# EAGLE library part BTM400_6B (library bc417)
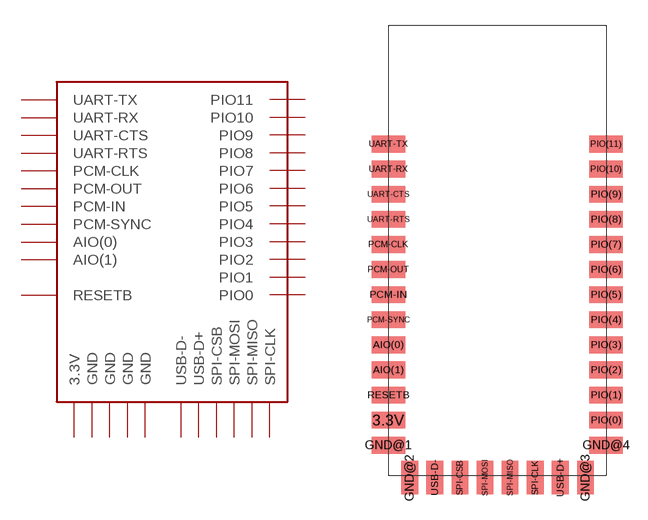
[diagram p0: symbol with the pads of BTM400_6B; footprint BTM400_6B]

Designator prefix -

## BTM400_6B  [BTM400_6B]
3.3V  3.3V  pwr
AIO(0)  AIO(0)
AIO(1)  AIO(1)
GND@1  GND  pwr
GND@2  GND  pwr
GND@3  GND  pwr
GND@4  GND  pwr
PCM-CLK  PCM-CLK
PCM-IN  PCM-IN
PCM-OUT  PCM-OUT
PCM-SYNC  PCM-SYNC
PIO(0)  PIO0
PIO(1)  PIO1
PIO(2)  PIO2
PIO(3)  PIO3
PIO(4)  PIO4
PIO(5)  PIO5
PIO(6)  PIO6
PIO(7)  PIO7
PIO(8)  PIO8
PIO(9)  PIO9
PIO(10)  PIO10
PIO(11)  PIO11
RESETB  RESETB
SPI-CLK  SPI-CLK
SPI-CSB  SPI-CSB
SPI-MISO  SPI-MISO
SPI-MOSI  SPI-MOSI
UART-CTS  UART-CTS
UART-RTS  UART-RTS
UART-RX  UART-RX
UART-TX  UART-TX
USB-D+  USB-D+
USB-D-  USB-D-

## Footprint BTM400_6B (pad centres in mm)
smd 2 x 1: 3.3V -6.5,-10.16; AIO(0) -6.5,-5.66; AIO(1) -6.5,-7.16; GND@1 -6.5,-11.66; GND@4 6.5,-11.66; PCM-CLK -6.5,0.34; PCM-IN -6.5,-2.66; PCM-OUT -6.5,-1.16; PCM-SYNC -6.5,-4.16; PIO(0) 6.5,-10.16; PIO(1) 6.5,-8.66; PIO(2) 6.5,-7.16; PIO(3) 6.5,-5.66; PIO(4) 6.5,-4.16; PIO(5) 6.5,-2.66; PIO(6) 6.5,-1.16; PIO(7) 6.5,0.34; PIO(8) 6.5,1.84; PIO(9) 6.5,3.34; PIO(10) 6.5,4.84; PIO(11) 6.5,6.34; RESETB -6.5,-8.66; UART-CTS -6.5,3.34; UART-RTS -6.5,1.84; UART-RX -6.5,4.84; UART-TX -6.5,6.34
smd 1 x 2: GND@2 -5.23,-13.6; GND@3 5.27,-13.6; SPI-CLK 2.27,-13.6; SPI-CSB -2.23,-13.6; SPI-MISO 0.77,-13.6; SPI-MOSI -0.73,-13.6; USB-D+ 3.77,-13.6; USB-D- -3.73,-13.6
